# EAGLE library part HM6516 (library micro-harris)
MICROCONTROLLER/MEMORY DEVICE
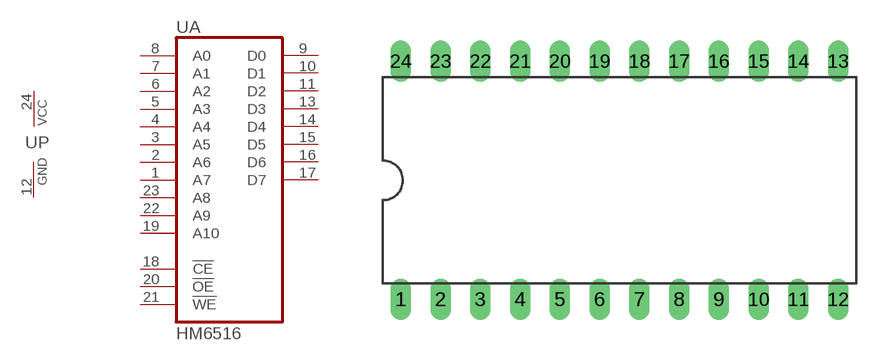
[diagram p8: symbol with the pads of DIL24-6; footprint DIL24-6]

Designator prefix U; gates A=HM6516 P=PWRN

## HM6516 (OC_FARNELL: unknown; OC_NEWARK: unknown)  [DIL24-6]
1  A:A7  in
2  A:A6  in
3  A:A5  in
4  A:A4  in
5  A:A3  in
6  A:A2  in
7  A:A1  in
8  A:A0  in
9  A:D0
10  A:D1
11  A:D2
12  P:GND  pwr
13  A:D3
14  A:D4
15  A:D5
16  A:D6
17  A:D7
18  A:!CE  in
19  A:A10  in
20  A:!OE  in
21  A:!WE  in
22  A:A9  in
23  A:A8  in
24  P:VCC  pwr

## Footprint DIL24-6 (pad centres in mm)
Dual In Line Package 0.6 inch
drill 0.813 long: 1 -13.97,-7.62; 2 -11.43,-7.62; 3 -8.89,-7.62; 4 -6.35,-7.62; 5 -3.81,-7.62; 6 -1.27,-7.62; 7 1.27,-7.62; 8 3.81,-7.62; 9 6.35,-7.62; 10 8.89,-7.62; 11 11.43,-7.62; 12 13.97,-7.62; 13 13.97,7.62; 14 11.43,7.62; 15 8.89,7.62; 16 6.35,7.62; 17 3.81,7.62; 18 1.27,7.62; 19 -1.27,7.62; 20 -3.81,7.62; 21 -6.35,7.62; 22 -8.89,7.62; 23 -11.43,7.62; 24 -13.97,7.62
